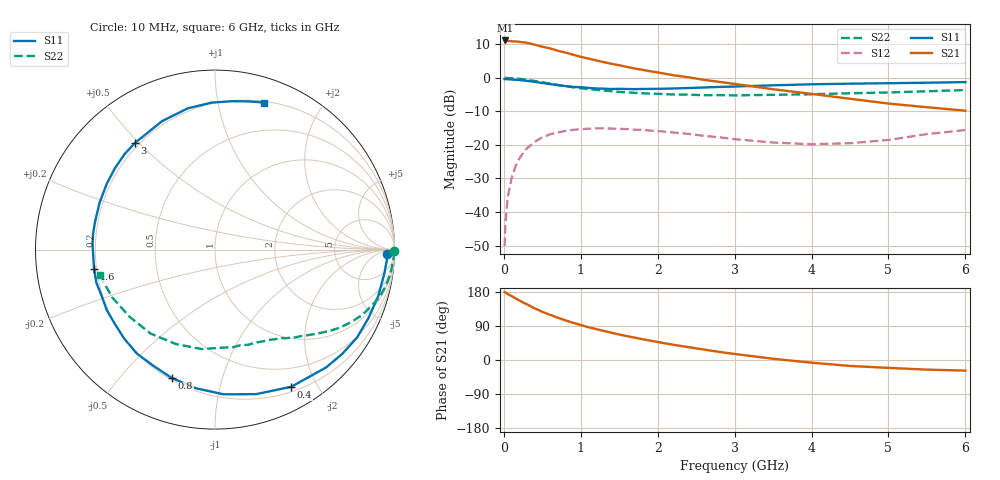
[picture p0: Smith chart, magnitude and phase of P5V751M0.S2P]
! SIEMENS Small Signal Semiconductors
! BFP183
! Si NPN RF Bipolar Junction Transistor in SOT143
! VCE = 0.75 V  IC = 1 mA
! Common Emitter S-Parameters:  March  1996
# GHz  S  MA  R  50
!  f  S11  S21  S12  S22
! GHz  MAG  ANG  MAG  ANG  MAG  ANG  MAG  ANG
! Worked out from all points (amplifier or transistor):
!   36 points, 10 MHz to 6 GHz, reference 50 ohm
!   highest |S21| = 11.2 dB at 20 MHz (marker M1)
!   |S21| within 3 dB of that: start of sweep to 692.3 MHz
!   unconditionally stable (mu >= 1): 2.363 GHz to end of sweep
!   at 250 MHz: K = 0.11, MSG = 16.5 dB, |S12| = -22.4 dB
!   at 1.4 GHz: K = 0.59, MSG = 9.6 dB, |S12| = -15.1 dB
!   at 6 GHz: K = 1.28, MAG = -0.3 dB, |S12| = -15.6 dB
!   S11 on the Smith chart (normalised r, x): 10 MHz: 34, -21; 400 MHz: 0.26, -1.67; 800 MHz: 0.21, -0.70; 1.6 GHz: 0.19, -0.08; 3 GHz: 0.18, +0.49; 6 GHz: 0.21, +1.37
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0.01  0.958 -1.5  3.551 179.2  0.0031 85.6  0.9999 -0.6
0.02  0.9597 -3.3  3.61 178.4  0.0066 83.5  0.9993 -1.3
0.05  0.9528 -8.1  3.562 174.3  0.0163 86.2  0.9944 -3.2
0.1  0.9456 -15.9  3.506 168.7  0.0318 79.3  0.9888 -6.5
0.15  0.9364 -24.1  3.486 163.0  0.0473 75.3  0.9802 -9.8
0.25  0.9165 -39.4  3.386 151.8  0.0762 66.0  0.9555 -15.8
0.3  0.9024 -46.7  3.332 147.1  0.0889 61.7  0.9352 -18.6
0.4  0.8743 -60.9  3.125 136.5  0.1112 53.4  0.8993 -23.7
0.5  0.8375 -74.1  2.913 127.3  0.1297 45.8  0.8591 -28.1
0.6  0.8078 -86.6  2.75 119.2  0.1438 39.1  0.8203 -32.0
0.8  0.7553 -108.4  2.386 104.5  0.1616 28.0  0.7509 -38.1
0.9  0.733 -117.8  2.211 98.3  0.1681 23.3  0.7242 -40.6
1.1  0.7086 -135.5  1.941 86.5  0.1748 15.0  0.6793 -45.2
1.4  0.6821 -157.8  1.62 71.9  0.1757 4.9  0.6322 -51.4
1.6  0.6827 -170.9  1.458 63.0  0.1725 0.0  0.6087 -54.7
1.9  0.6848 172.4  1.256 51.2  0.1639 -6.2  0.5831 -60.5
2.2  0.6941 157.8  1.097 40.2  0.1536 -10.6  0.5655 -66.4
3  0.7429 126.8  0.812 15.9  0.1219 -14.8  0.548 -84.8
3.5  0.7742 112.4  0.677 3.3  0.1087 -10.4  0.5589 -97.5
4.5  0.8192 91.3  0.488 -15.7  0.1062 6.4  0.5897 -127.5
5.5  0.8468 77.2  0.365 -25.4  0.1453 15.8  0.6311 -154.9
6  0.8639 71.4  0.324 -28.0  0.1664 13.7  0.658 -167.4
